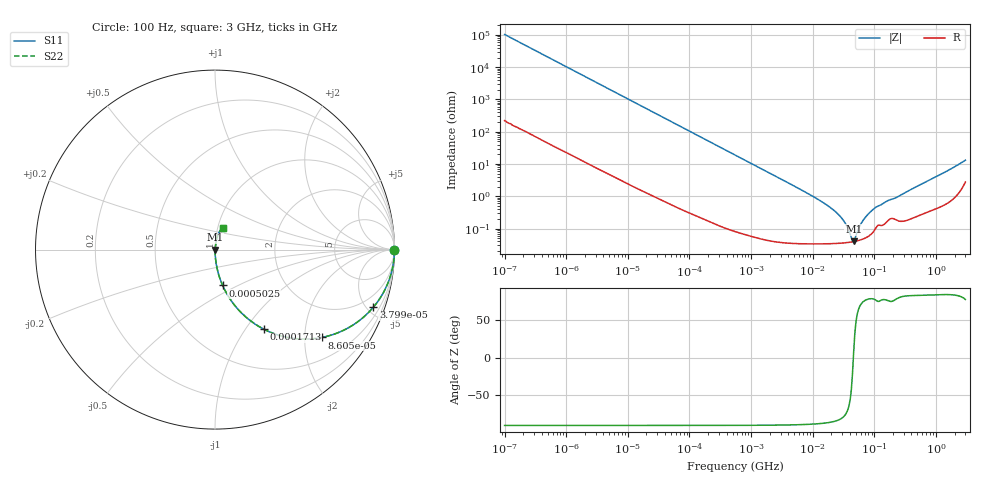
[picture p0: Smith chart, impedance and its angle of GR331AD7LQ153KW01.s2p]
!Murata Part Number: GR331AD7LQ153KW01
!These Parameters are Measured in Series Mode Connection
!Data Generated on Jun 10, 2025
!  o--ll--o
!Port1  Port2
!  o------o
!Operation Temp=25[degC], DC Bias Voltage=0[V]
!Freq. Start=100[Hz] Stop=3[GHz] 401[Steps]
# Hz S RI R 50
!Freq.(Hz) S11(Real) S11(Imag) S21(Real) S21(Imag) S12(Real) S12(Imag) S22(Real) S22(Imag)
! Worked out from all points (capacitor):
!   401 points, 100 Hz to 3 GHz, reference 50 ohm
!   read as one part in series: C = 15.4 nF near 109 Hz
!   lowest |Z| = 39.8 mohm at 46.12 MHz (marker M1)
!   series resonance near 45.61 MHz, so ESL is about 790 pH
!   S11 on the Smith chart (normalised r, x): 100 Hz: open; 37.98 kHz: 1.01, -5.49; 86.05 kHz: 1.01, -2.43; 171.3 kHz: 1.00, -1.22; 502.5 kHz: 1.00, -0.42; 3 GHz: 1.06, +0.26
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100  1 -0.000967  3e-06 0.000967  3e-06 0.000967  1 -0.000967
1788  0.9997 -0.0172  0.000334 0.0172  0.000334 0.0172  0.9997 -0.0172
9582  0.9914 -0.0912  0.00861 0.0912  0.00861 0.0912  0.9914 -0.0912
31977  0.9135 -0.2798  0.0865 0.2798  0.0865 0.2798  0.9135 -0.2798
37985  0.8823 -0.3209  0.1177 0.3209  0.1177 0.3209  0.8823 -0.3209
86054  0.5955 -0.4894  0.4045 0.4894  0.4045 0.4894  0.5955 -0.4894
171338  0.2721 -0.4435  0.7279 0.4435  0.7279 0.4435  0.2721 -0.4435
287190  0.1181 -0.321  0.8819 0.321  0.8819 0.321  0.1181 -0.321
502545  0.0424 -0.1995  0.9576 0.1995  0.9576 0.1995  0.0424 -0.1995
547723  0.036 -0.1843  0.964 0.1843  0.964 0.1843  0.036 -0.1843
1750920  0.00401 -0.0596  0.996 0.0596  0.996 0.0596  0.00401 -0.0596
9794414  0.000439 -0.0102  0.9996 0.0102  0.9996 0.0102  0.000439 -0.0102
1.789277e7  0.000362 -0.00497  0.9996 0.00497  0.9996 0.00497  0.000362 -0.00497
2.635803e7  0.000356 -0.00266  0.9996 0.00266  0.9996 0.00266  0.000356 -0.00266
3.268714e7  0.000362 -0.00157  0.9996 0.00157  0.9996 0.00157  0.000362 -0.00157
4.231884e7  0.000383 -0.000346  0.9996 0.000346  0.9996 0.000346  0.000383 -0.000346
4.612319e7  0.000394 5.24e-05  0.9996 -5.24e-05  0.9996 -5.24e-05  0.000394 5.24e-05
6.234031e7  0.00046 0.00148  0.9995 -0.00148  0.9995 -0.00148  0.00046 0.00148
7.730952e7  0.000558 0.00259  0.9994 -0.00259  0.9994 -0.00259  0.000558 0.00259
1.044919e8  0.00102 0.00438  0.999 -0.00438  0.999 -0.00438  0.00102 0.00438
1.751444e8  0.00196 0.0074  0.998 -0.0074  0.998 -0.0074  0.00196 0.0074
3e9  0.0418 0.1197  0.9582 -0.1197  0.9582 -0.1197  0.0418 0.1197
